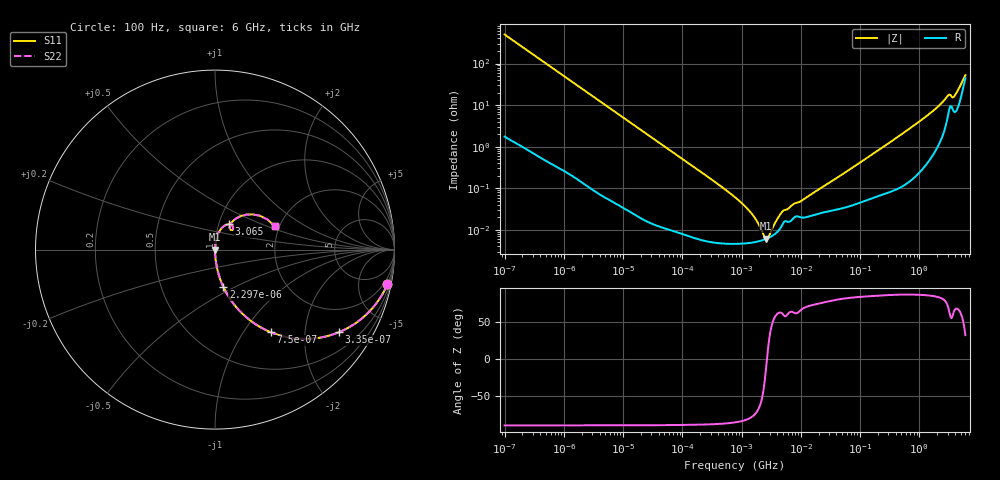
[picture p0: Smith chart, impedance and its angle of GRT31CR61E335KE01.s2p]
!Murata Part Number: GRT31CR61E335KE01
!These Parameters are Measured in Series Mode Connection
!Data Generated on Jun 19, 2026
!  o--ll--o
!Port1  Port2
!  o------o
!Operation Temp=25[degC], DC Bias Voltage=0[V]
!Freq. Start=100[Hz] Stop=6[GHz] 401[Steps]
# Hz S RI R 50
!Freq.(Hz) S11(Real) S11(Imag) S21(Real) S21(Imag) S12(Real) S12(Imag) S22(Real) S22(Imag)
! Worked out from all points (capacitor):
!   401 points, 100 Hz to 6 GHz, reference 50 ohm
!   read as one part in series: C = 3.19 uF near 109 Hz
!   lowest |Z| = 6.21 mohm at 2.595 MHz (marker M1)
!   series resonance near 2.685 MHz, so ESL is about 1.1 nH
!   S11 on the Smith chart (normalised r, x): 100 Hz: 1, -10; 335 Hz: 1.01, -2.99; 750 Hz: 1.01, -1.34; 2.297 kHz: 1.00, -0.44; 3.065 GHz: 1.12, +0.32; 6 GHz: 1.89, +0.56
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100  0.9608 -0.1924  0.0392 0.1924  0.0392 0.1924  0.9608 -0.1924
196  0.866 -0.3387  0.134 0.3387  0.134 0.3387  0.866 -0.3387
335  0.6898 -0.4604  0.3102 0.4604  0.3102 0.4604  0.6898 -0.4604
750  0.3099 -0.46  0.6901 0.46  0.6901 0.46  0.3099 -0.46
1227  0.1449 -0.3493  0.8551 0.3493  0.8551 0.3493  0.1449 -0.3493
2008  0.0603 -0.2352  0.9397 0.2352  0.9397 0.2352  0.0603 -0.2352
2297  0.0469 -0.2087  0.9531 0.2087  0.9531 0.2087  0.0469 -0.2087
7358  0.00513 -0.0683  0.9949 0.0683  0.9949 0.0683  0.00513 -0.0683
40335  0.00028 -0.0126  0.9997 0.0126  0.9997 0.0126  0.00028 -0.0126
774597  4.64e-05 -0.000608  1 0.000608  1 0.000608  4.64e-05 -0.000608
1386327  4.87e-05 -0.000272  1 0.000272  1 0.000272  4.87e-05 -0.000272
2169299  5.55e-05 -8.21e-05  0.9999 8.21e-05  0.9999 8.21e-05  5.55e-05 -8.21e-05
2594782  6.07e-05 -1.3e-05  0.9999 1.3e-05  0.9999 1.3e-05  6.07e-05 -1.3e-05
3245845  7.1e-05 7.35e-05  0.9999 -7.35e-05  0.9999 -7.35e-05  7.1e-05 7.35e-05
5079039  0.000148 0.000252  0.9999 -0.000252  0.9999 -0.000252  0.000148 0.000252
1.555665e7  0.000223 0.000712  0.9998 -0.000712  0.9998 -0.000712  0.000223 0.000712
3.124326e8  0.000956 0.0124  0.999 -0.0124  0.999 -0.0124  0.000956 0.0124
1.431855e9  0.00783 0.0585  0.9922 -0.0585  0.9922 -0.0585  0.00783 0.0585
3.065283e9  0.0764 0.1407  0.9236 -0.1407  0.9236 -0.1407  0.0764 0.1407
3.8344e9  0.0815 0.1223  0.9185 -0.1223  0.9185 -0.1223  0.0815 0.1223
5.016141e9  0.1747 0.1949  0.8253 -0.1949  0.8253 -0.1949  0.1747 0.1949
6e9  0.3334 0.1292  0.6666 -0.1292  0.6666 -0.1292  0.3334 0.1292
